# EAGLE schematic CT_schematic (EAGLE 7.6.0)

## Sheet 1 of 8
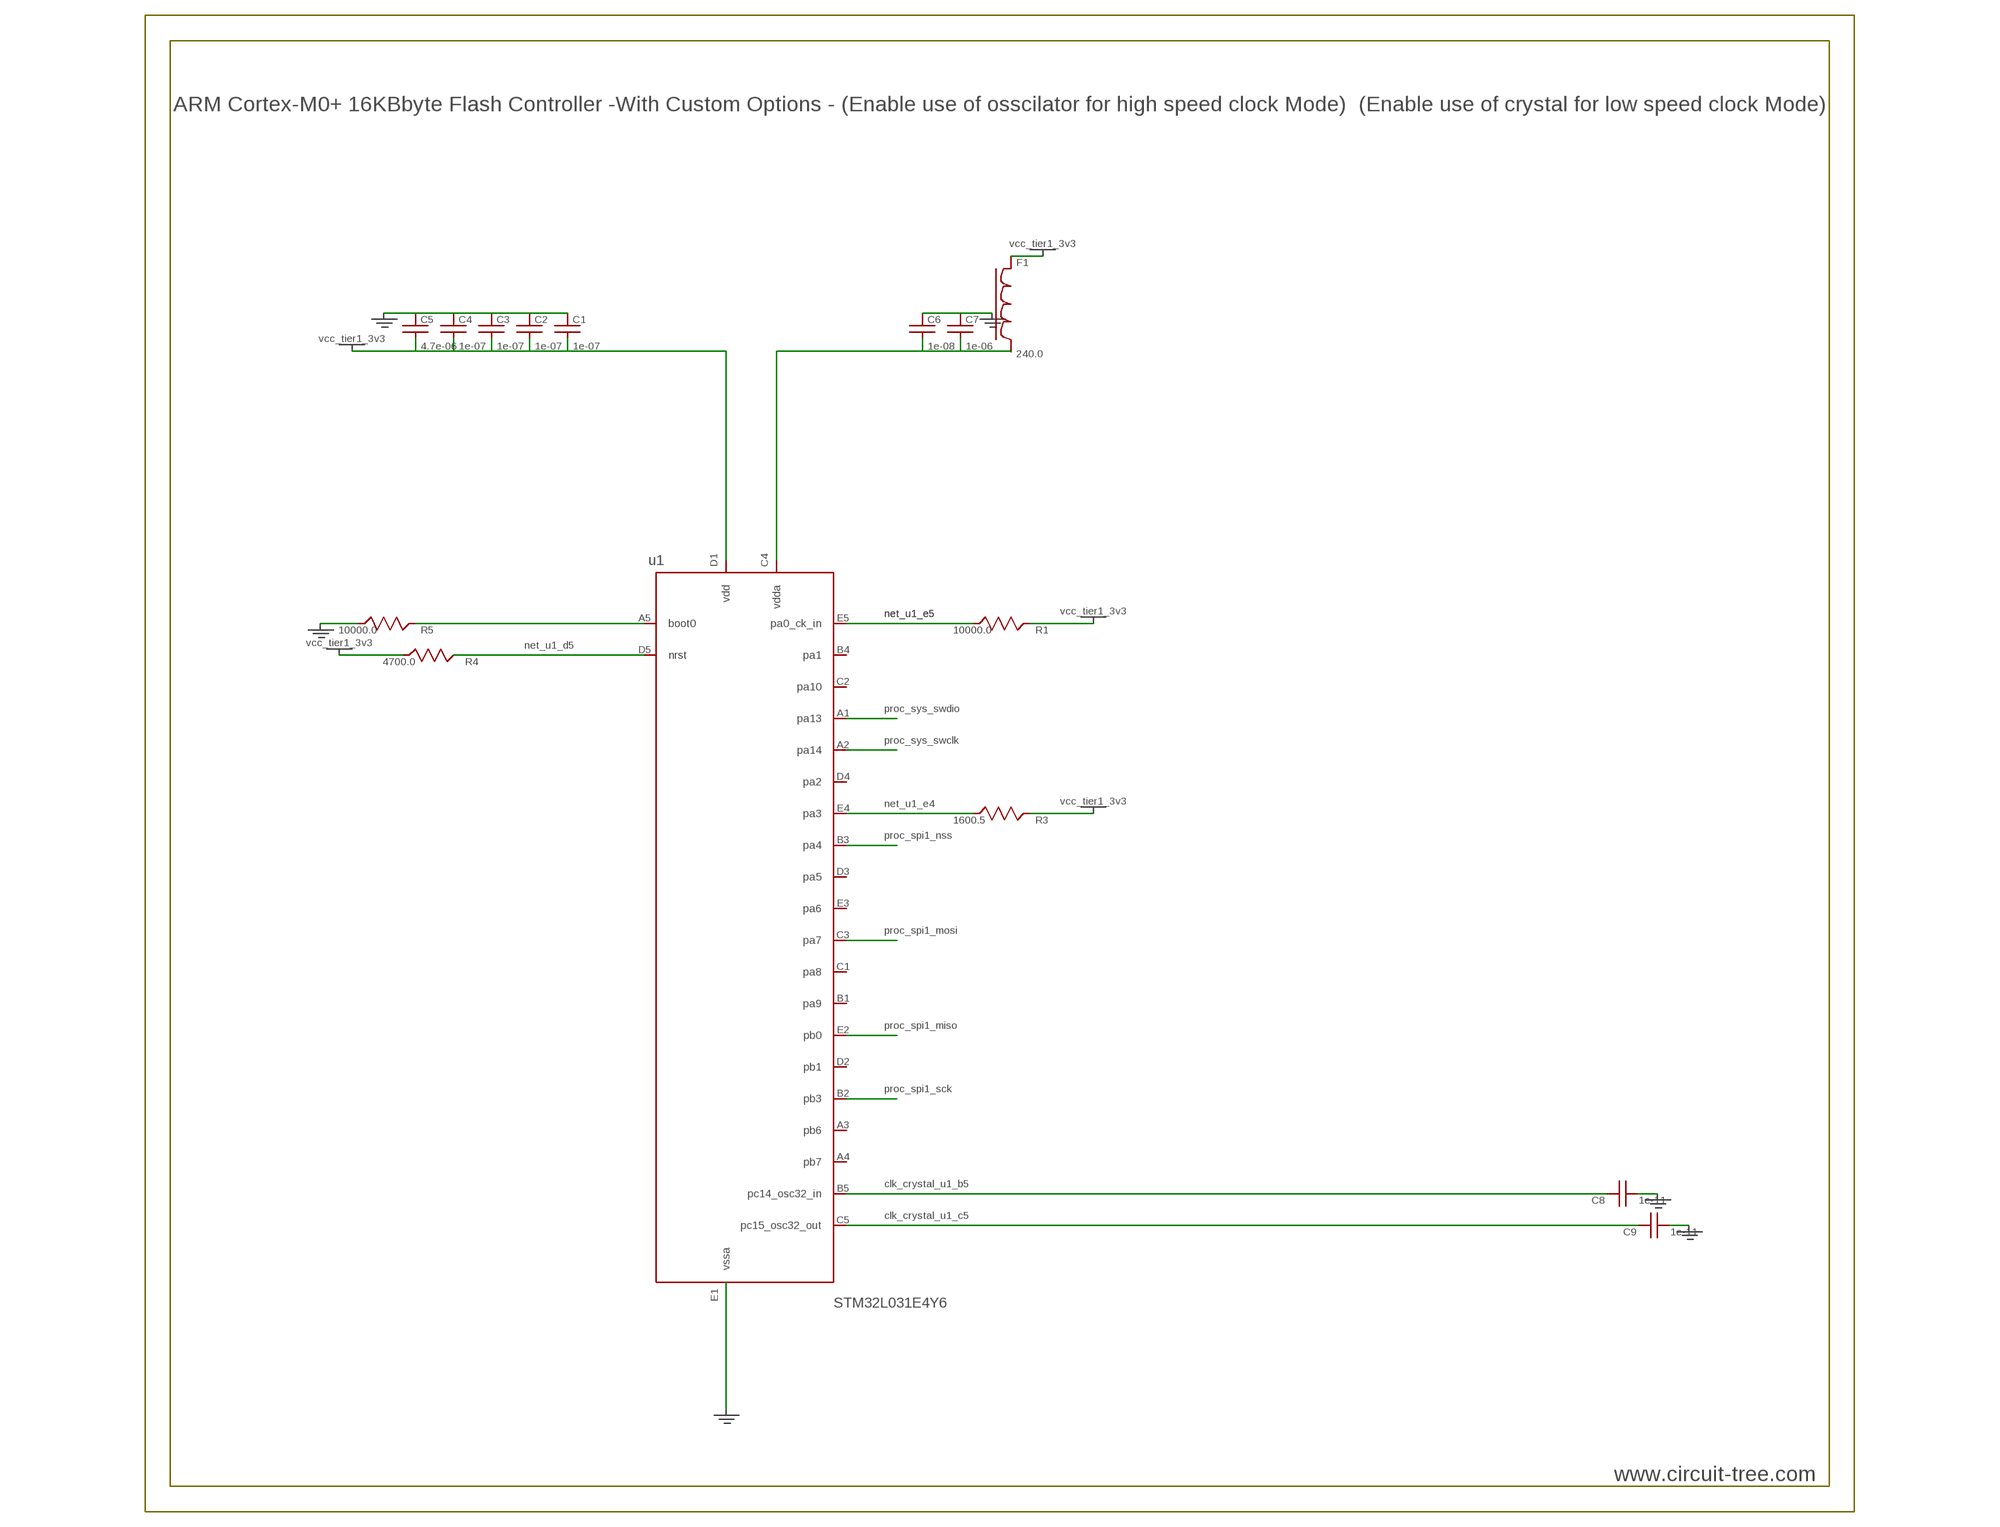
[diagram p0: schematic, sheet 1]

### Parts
C1  1e-07  06035C104K4Z2A  [C0603]
C2  1e-07  06035C104K4Z2A  [C0603]
C3  1e-07  06035C104K4Z2A  [C0603]
C4  1e-07  06035C104K4Z2A  [C0603]
C5  4.7e-06  GRM188R6YA475KE15D  [C0603]
C6  1e-08  06035C103K4Z2A  [C0603]
C7  1e-06  c0603c105k3ractu  [C0603]
C8  1e-11  C0402C100K3GACTU  [C0402]
C9  1e-11  C0402C100K3GACTU  [C0402]
F1  240.0  z0603c241asmst  [L0603]
R1  10000.0  RC0603JR-0710KL  [R0603]
R3  1600.5  R3  [R0603]
R4  4700.0  RC0603JR-074K7L  [R0603]
R5  10000.0  RC0603JR-0710KL  [R0603]
u1  STM32L031E4Y6  [WLCSP25]

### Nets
clk_crystal_u1_b5: C8.1 u1.B5(pc14_osc32_in) ; also sheet 4
clk_crystal_u1_c5: C9.1 u1.C5(pc15_osc32_out) ; also sheet 4
gnd: C1.2 C2.2 C3.2 C4.2 C5.2 C6.2 C7.2 C8.2 C9.2 R5.2 u1.E1(vssa) ; also sheet 2,3,4,5,6,7,8
net_u1_a5: R5.1 u1.A5(boot0)
net_u1_c4: C6.1 C7.1 F1.1 u1.C4(vdda)
net_u1_d5: R4.1 u1.D5(nrst) ; also sheet 8
net_u1_e4: R3.1 u1.E4(pa3) ; also sheet 8
net_u1_e5: R1.1 u1.E5(pa0_ck_in) ; also sheet 4,8
proc_spi1_miso: u1.E2(pb0) ; also sheet 3
proc_spi1_mosi: u1.C3(pa7) ; also sheet 3
proc_spi1_nss: u1.B3(pa4) ; also sheet 3
proc_spi1_sck: u1.B2(pb3) ; also sheet 3
proc_sys_swclk: u1.A2(pa14) ; also sheet 2
proc_sys_swdio: u1.A1(pa13) ; also sheet 2
vcc_tier1_3v3: C1.1 C2.1 C3.1 C4.1 C5.1 F1.2 R1.2 R3.2 R4.2 u1.D1(vdd) ; also sheet 2,3,4,5,6,8
Unconnected: u1.A3(pb6) u1.A4(pb7) u1.B1(pa9) u1.B4(pa1) u1.C1(pa8) u1.C2(pa10) u1.D2(pb1) u1.D3(pa5) u1.D4(pa2) u1.E3(pa6)

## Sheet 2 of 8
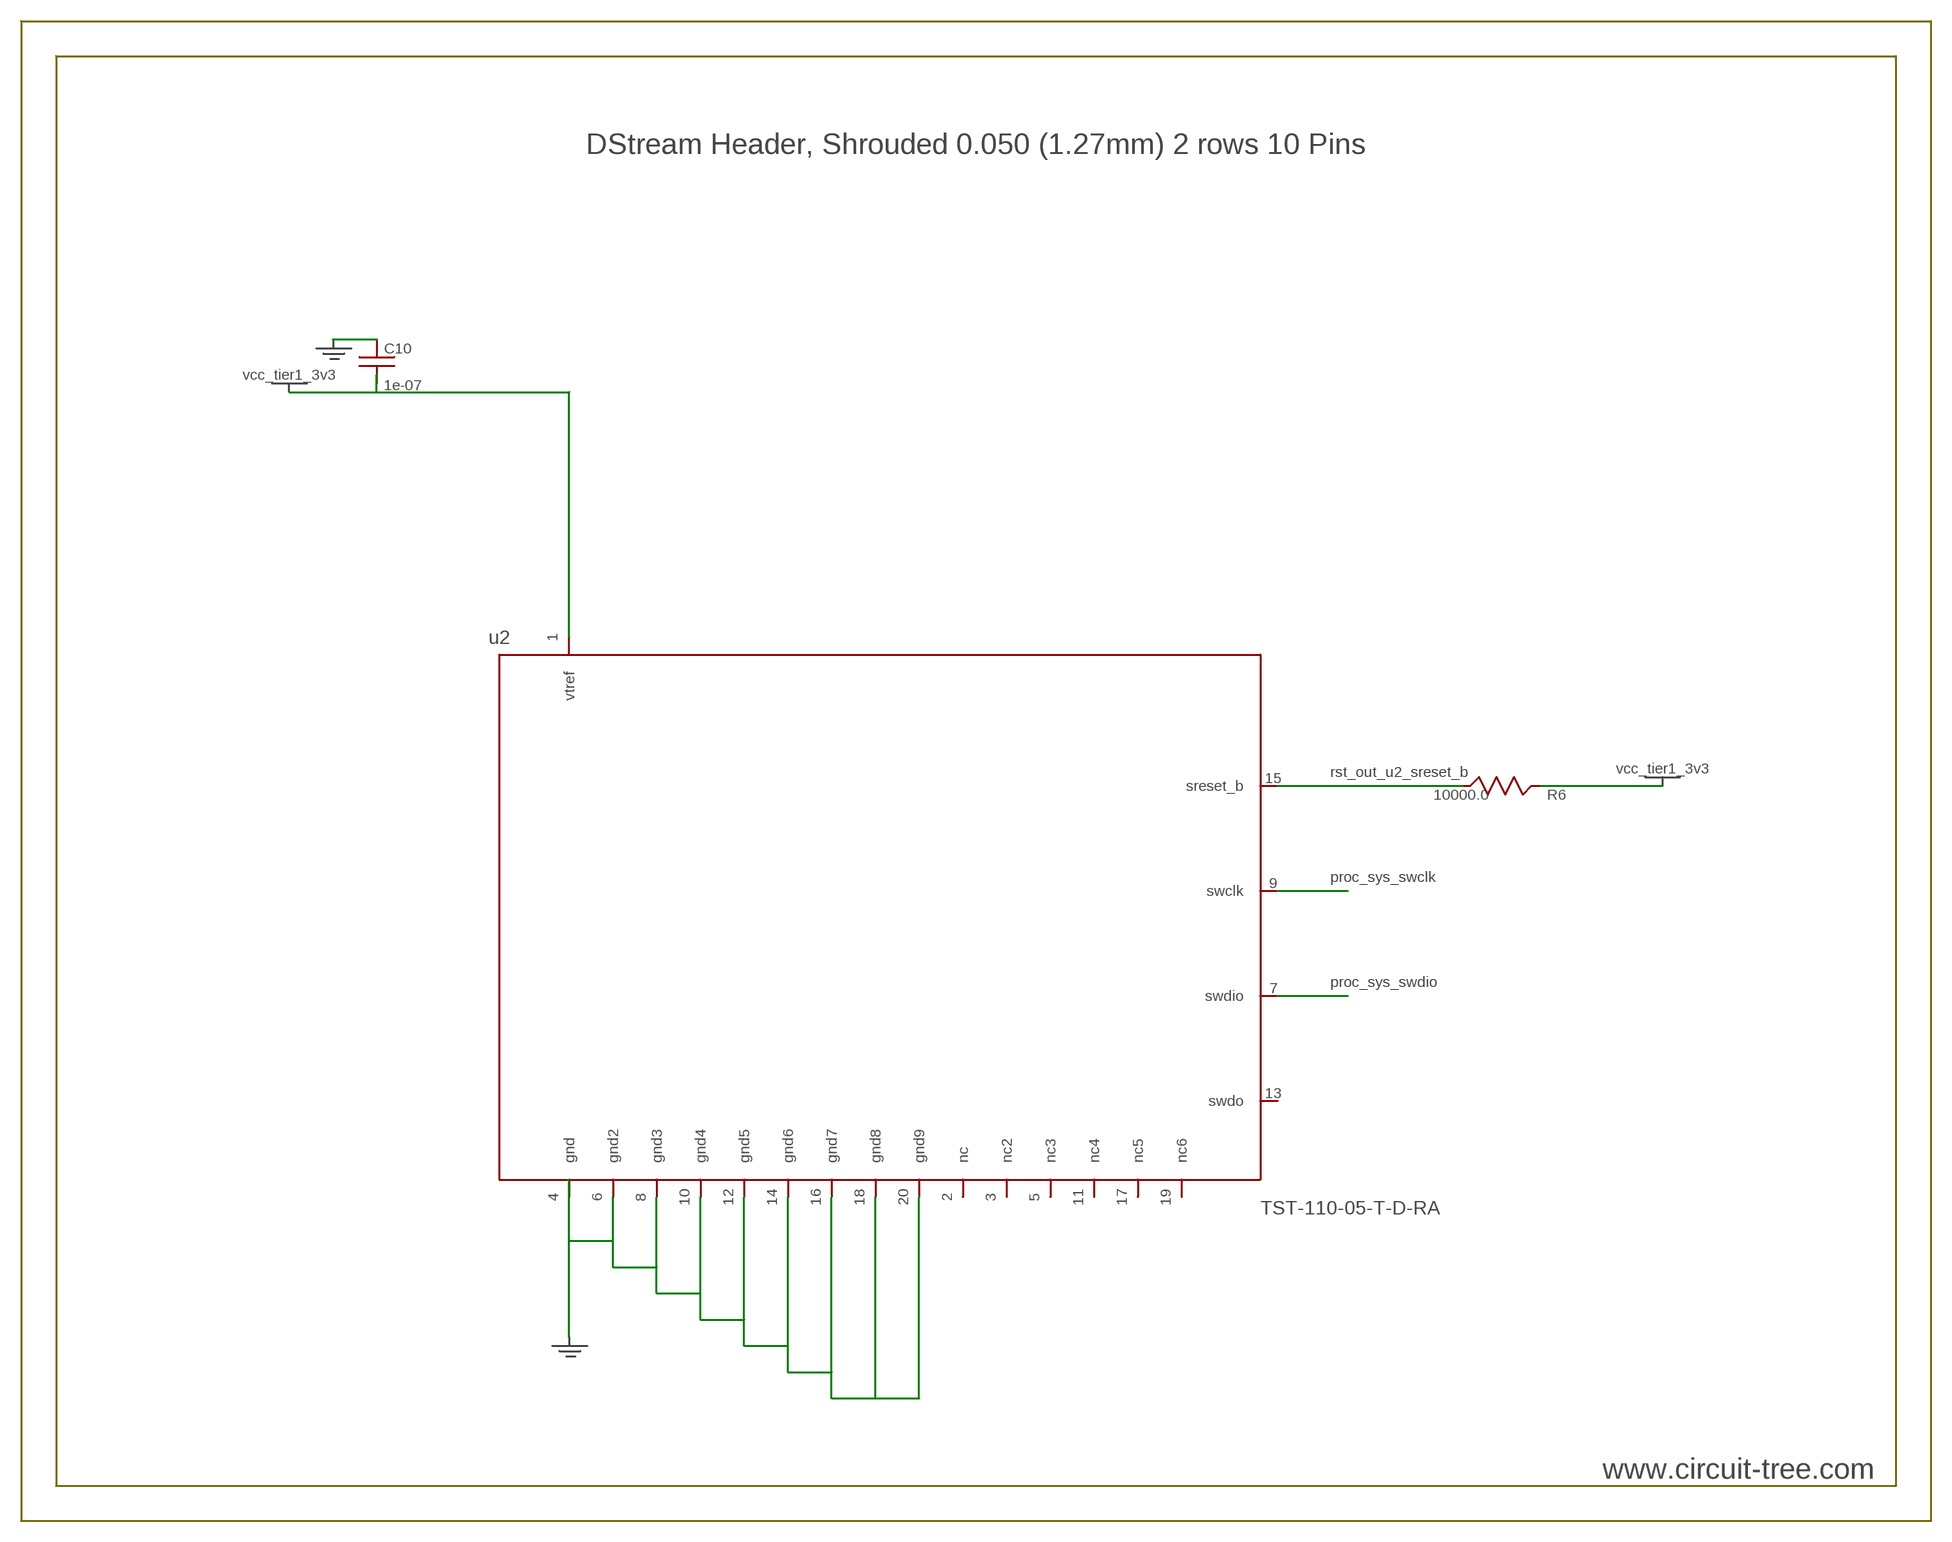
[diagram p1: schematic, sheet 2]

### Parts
C10  1e-07  c0402c104k3ractu  [C0402]
R6  10000.0  RC0603JR-0710KL  [R0603]
u2  TST-110-05-T-D-RA  [TST-110-05-T-D-RA]

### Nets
gnd: C10.2 u2.4(gnd) u2.6(gnd2) u2.8(gnd3) u2.10(gnd4) u2.12(gnd5) u2.14(gnd6) u2.16(gnd7) u2.18(gnd8) u2.20(gnd9) ; also sheet 1,3,4,5,6,7,8
proc_sys_swclk: u2.9(swclk) ; also sheet 1
proc_sys_swdio: u2.7(swdio) ; also sheet 1
rst_out_u2_sreset_b: R6.1 u2.15(sreset_b) ; also sheet 8
vcc_tier1_3v3: C10.1 R6.2 u2.1(vtref) ; also sheet 1,3,4,5,6,8
Unconnected: u2.2(nc) u2.3(nc2) u2.5(nc3) u2.11(nc4) u2.13(swdo) u2.17(nc5) u2.19(nc6)

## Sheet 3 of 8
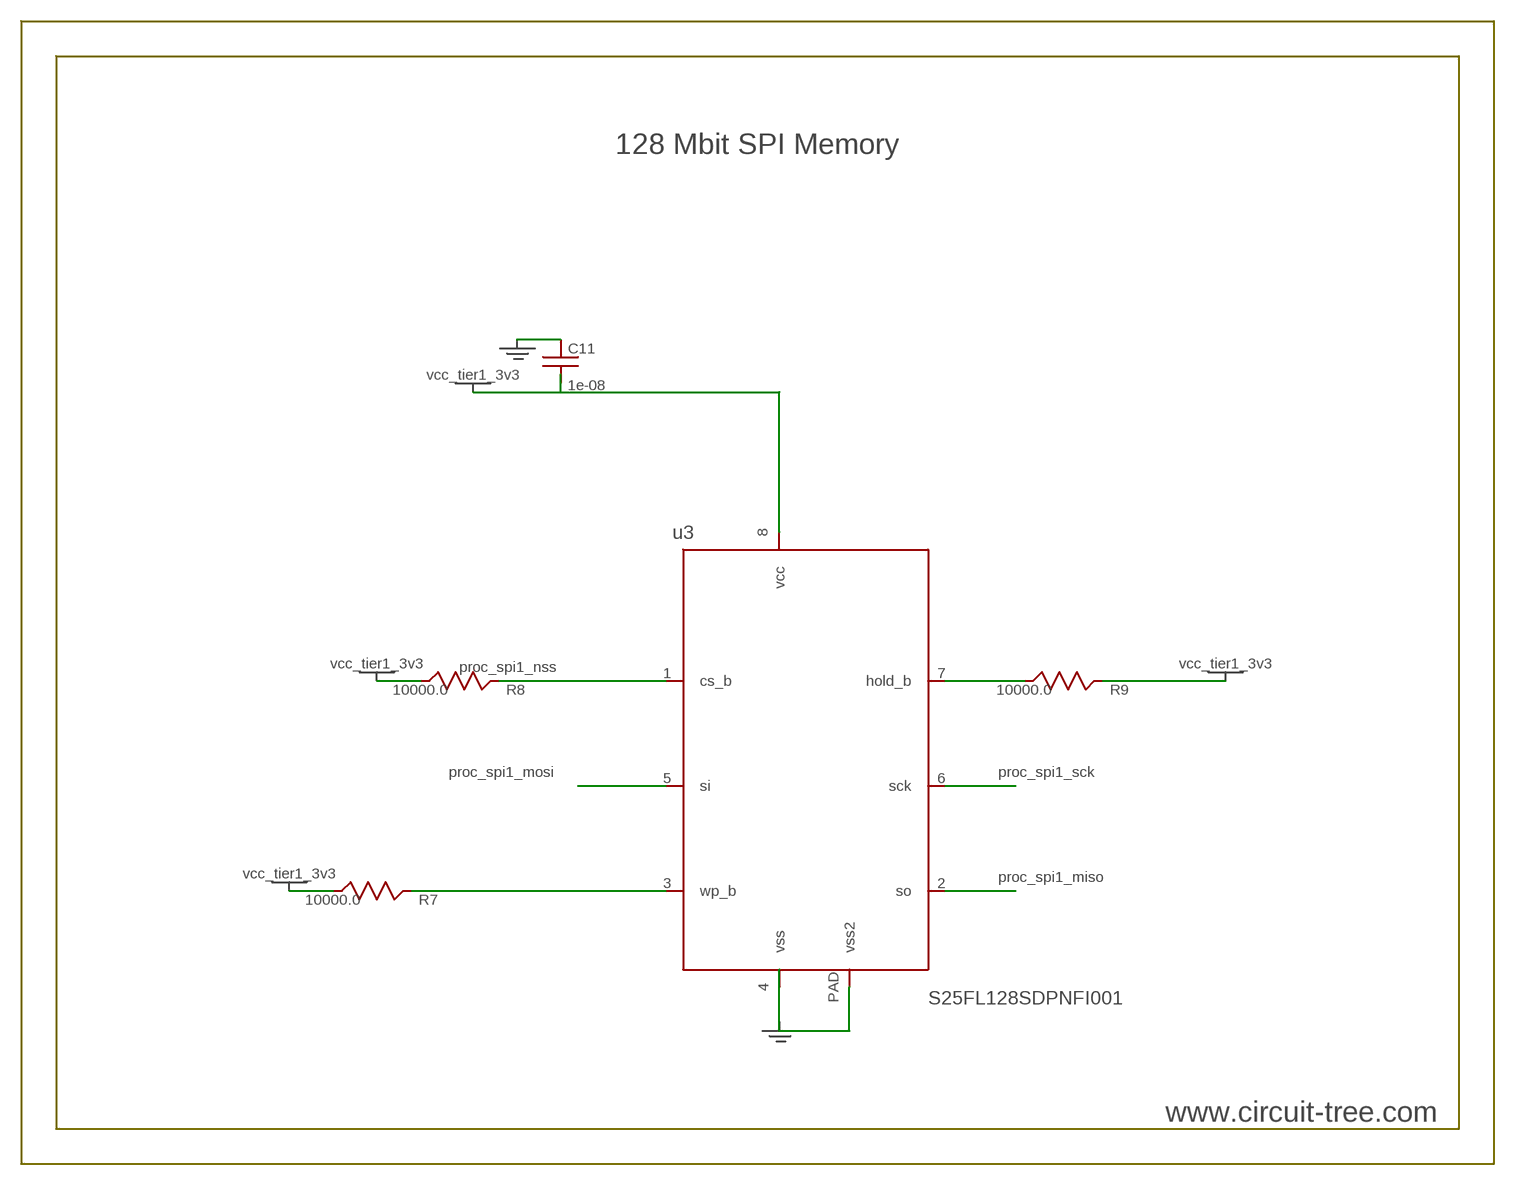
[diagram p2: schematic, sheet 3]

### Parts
C11  1e-08  c0402c103k3rac  [C0402]
R7  10000.0  RC0603JR-0710KL  [R0603]
R8  10000.0  RC0603JR-0710KL  [R0603]
R9  10000.0  RC0603JR-0710KL  [R0603]
u3  S25FL128SDPNFI001  [WNG008]

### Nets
gnd: C11.2 u3.4(vss) u3.PAD(vss2) ; also sheet 1,2,4,5,6,7,8
net_u3_3: R7.1 u3.3(wp_b)
net_u3_7: R9.1 u3.7(hold_b)
proc_spi1_miso: u3.2(so) ; also sheet 1
proc_spi1_mosi: u3.5(si) ; also sheet 1
proc_spi1_nss: R8.1 u3.1(cs_b) ; also sheet 1
proc_spi1_sck: u3.6(sck) ; also sheet 1
vcc_tier1_3v3: C11.1 R7.2 R8.2 R9.2 u3.8(vcc) ; also sheet 1,2,4,5,6,8

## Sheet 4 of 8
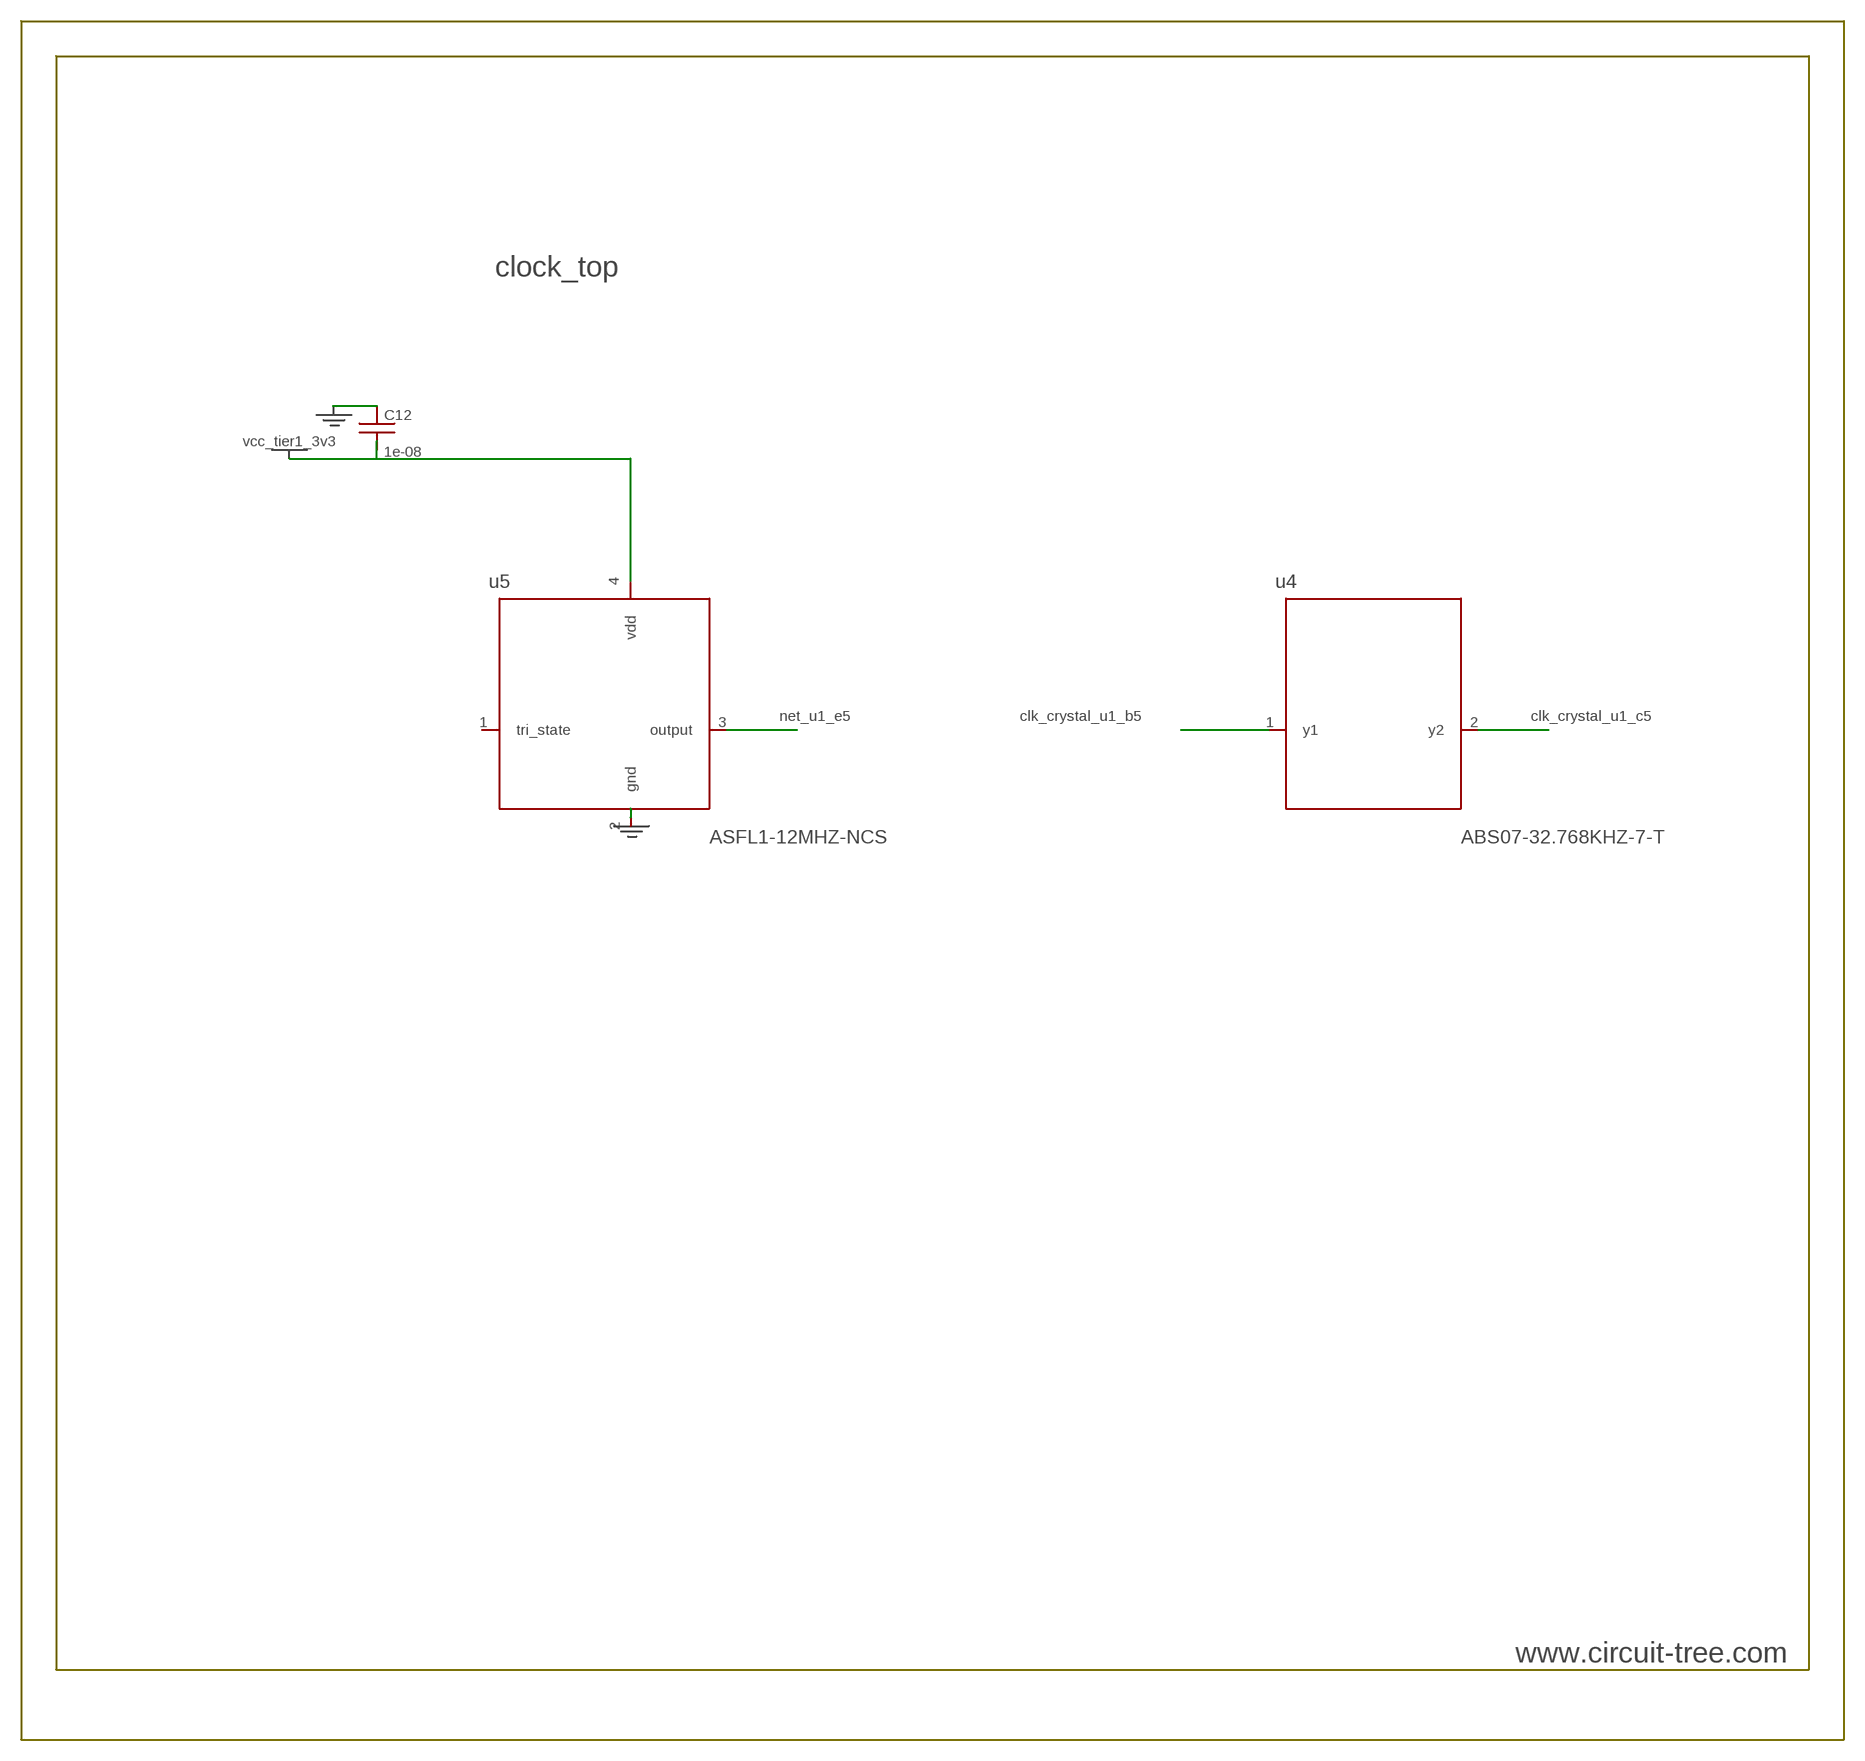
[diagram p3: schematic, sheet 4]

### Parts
C12  1e-08  c0402c103k3rac  [C0402]
u4  ABS07-32.768KHZ-7-T  [ABS07-32.768KHZ-7-T]
u5  ASFL1-12MHZ-NCS  [ASFL1]

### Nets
clk_crystal_u1_b5: u4.1(y1) ; also sheet 1
clk_crystal_u1_c5: u4.2(y2) ; also sheet 1
gnd: C12.2 u5.2(gnd) ; also sheet 1,2,3,5,6,7,8
net_u1_e5: u5.3(output) ; also sheet 1,8
vcc_tier1_3v3: C12.1 u5.4(vdd) ; also sheet 1,2,3,5,6,8
Unconnected: u5.1(tri_state)

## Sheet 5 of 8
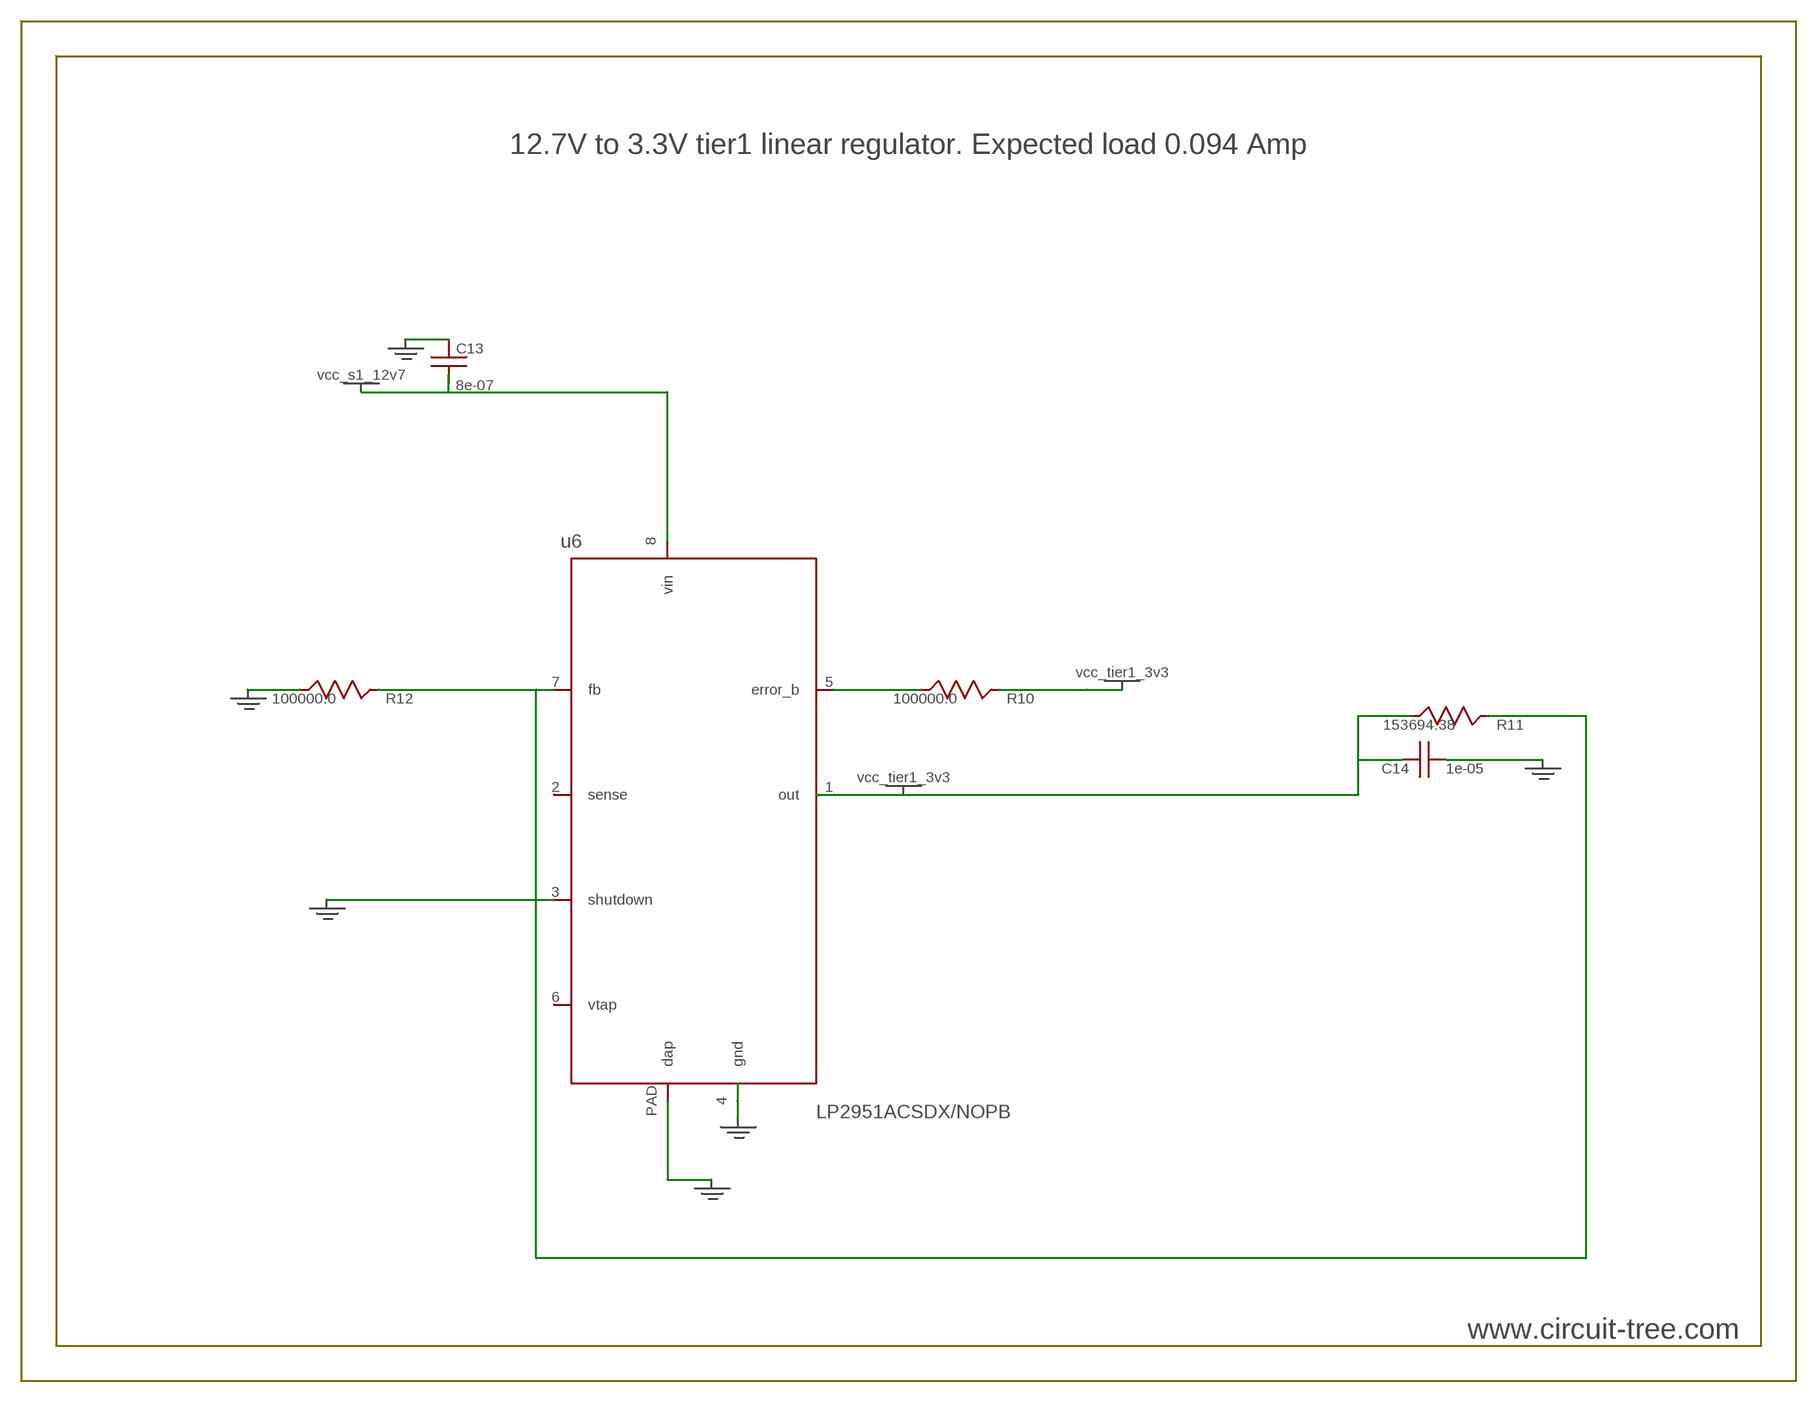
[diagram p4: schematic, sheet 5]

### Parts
C13  8e-07  C13  [R0603]
C14  1e-05  grm32DR61E106MA12L  [C1210]
R10  100000.0  RC0603JR-07100KL  [R0603]
R11  153694.38  R11  [R0603]
R12  100000.0  RC0603JR-07100KL  [R0603]
u6  LP2951ACSDX/NOPB  [WSON-8]

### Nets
gnd: C13.2 C14.2 R12.2 u6.3(shutdown) u6.4(gnd) u6.PAD(dap) ; also sheet 1,2,3,4,6,7,8
net_u6_5: R10.1 u6.5(error_b)
net_u6_7: R11.2 R12.1 u6.7(fb)
vcc_s1_12v7: C13.1 u6.8(vin) ; also sheet 7
vcc_tier1_3v3: c14.1 C14.1 r10.2 R10.2 r11.1 R11.1 u6.1(out) ; also sheet 1,2,3,4,6,8
Unconnected: u6.2(sense) u6.6(vtap)

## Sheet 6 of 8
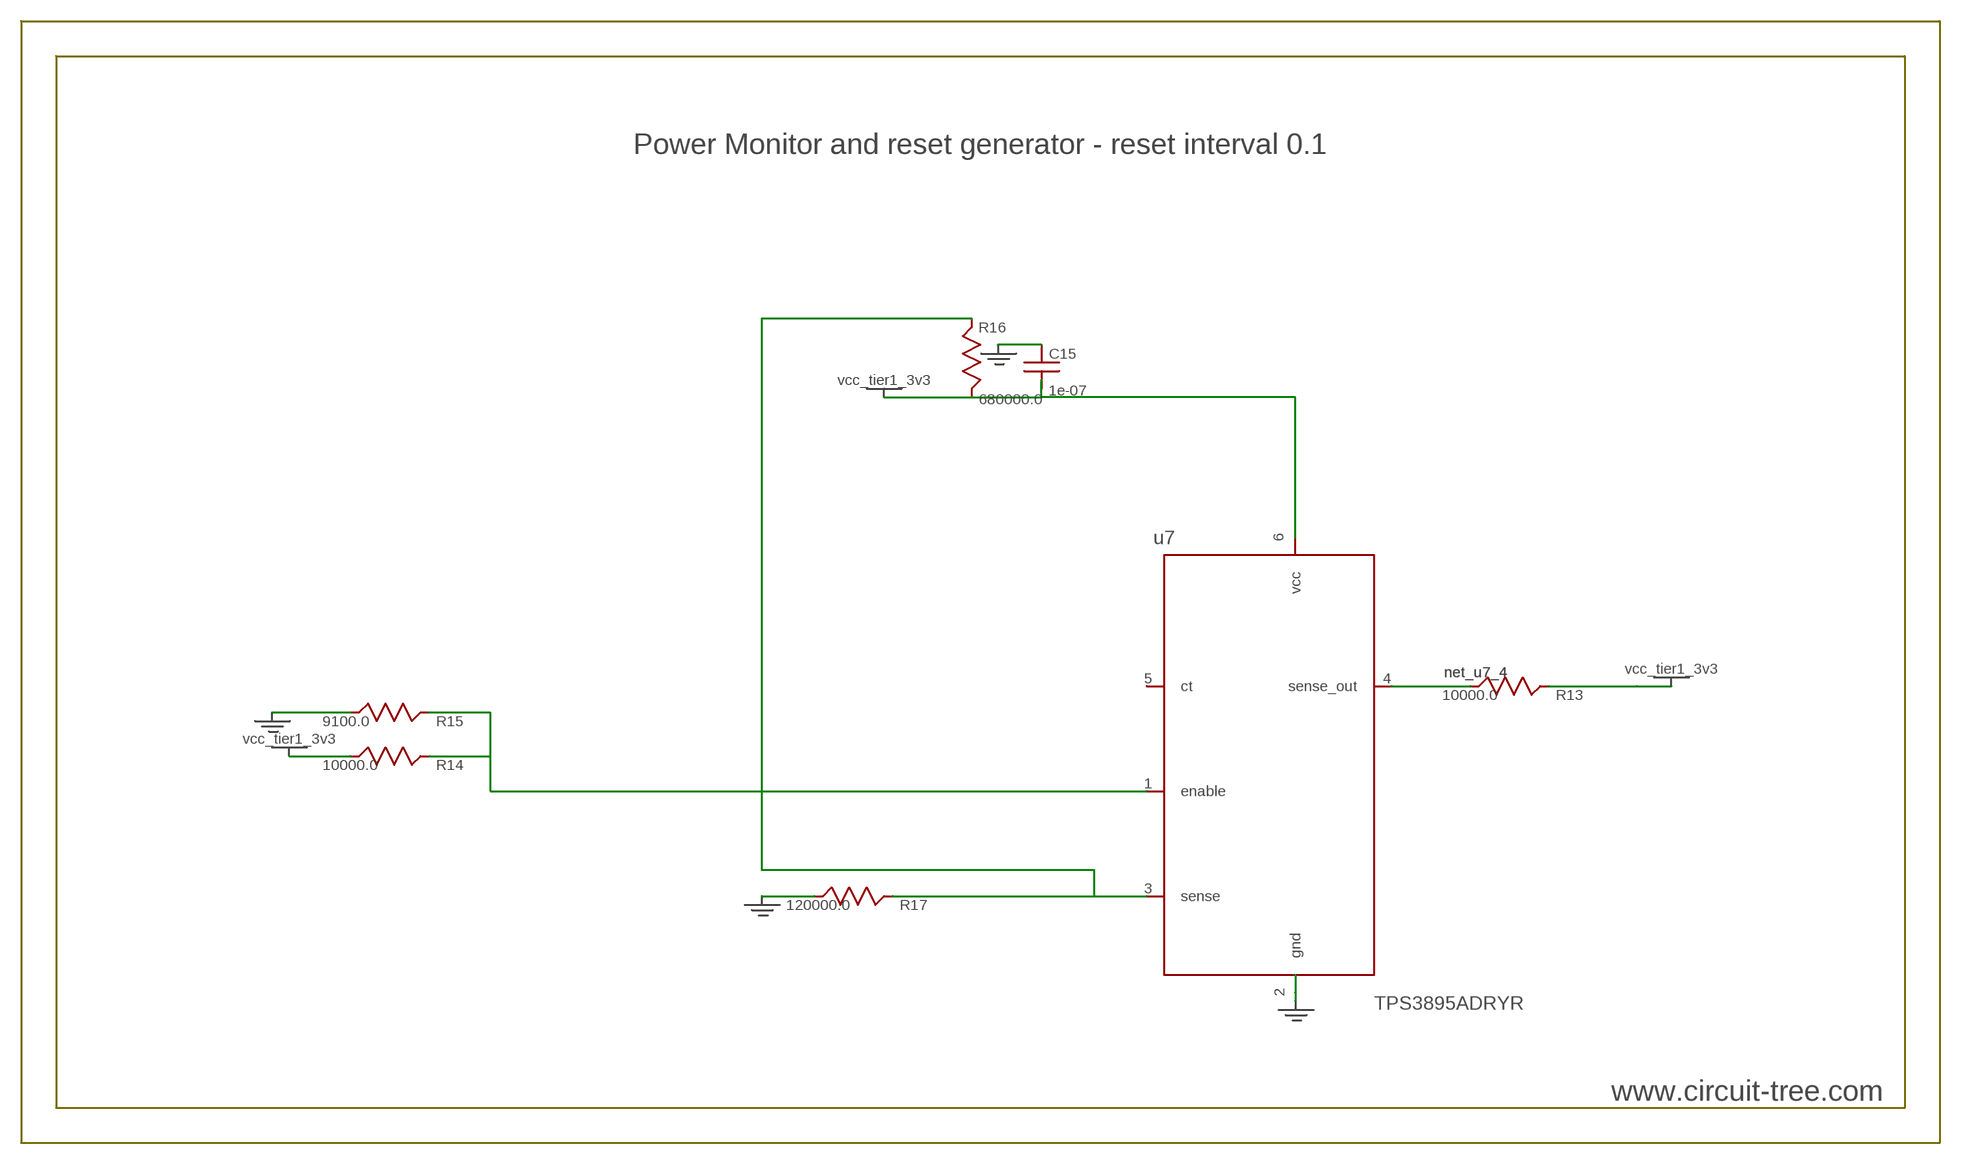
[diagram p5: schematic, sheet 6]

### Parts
C15  1e-07  c0402c104k3ractu  [C0402]
R13  10000.0  RC0603JR-0710KL  [R0603]
R14  10000.0  RC0603JR-0710KL  [R0603]
R15  9100.0  RC0603JR-079K1L  [R0603]
R16  680000.0  RC0603JR-07680KL  [R0603]
R17  120000.0  RC0603JR-07120KL  [R0603]
u7  TPS3895ADRYR  [SON-6]

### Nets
gnd: C15.2 R15.2 R17.2 u7.2(gnd) ; also sheet 1,2,3,4,5,7,8
net_u7_1: R14.1 R15.1 u7.1(enable)
net_u7_3: R16.2 R17.1 u7.3(sense)
net_u7_4: R13.1 u7.4(sense_out) ; also sheet 8
vcc_tier1_3v3: C15.1 R13.2 R14.2 R16.1 u7.6(vcc) ; also sheet 1,2,3,4,5,8
Unconnected: u7.5(ct)

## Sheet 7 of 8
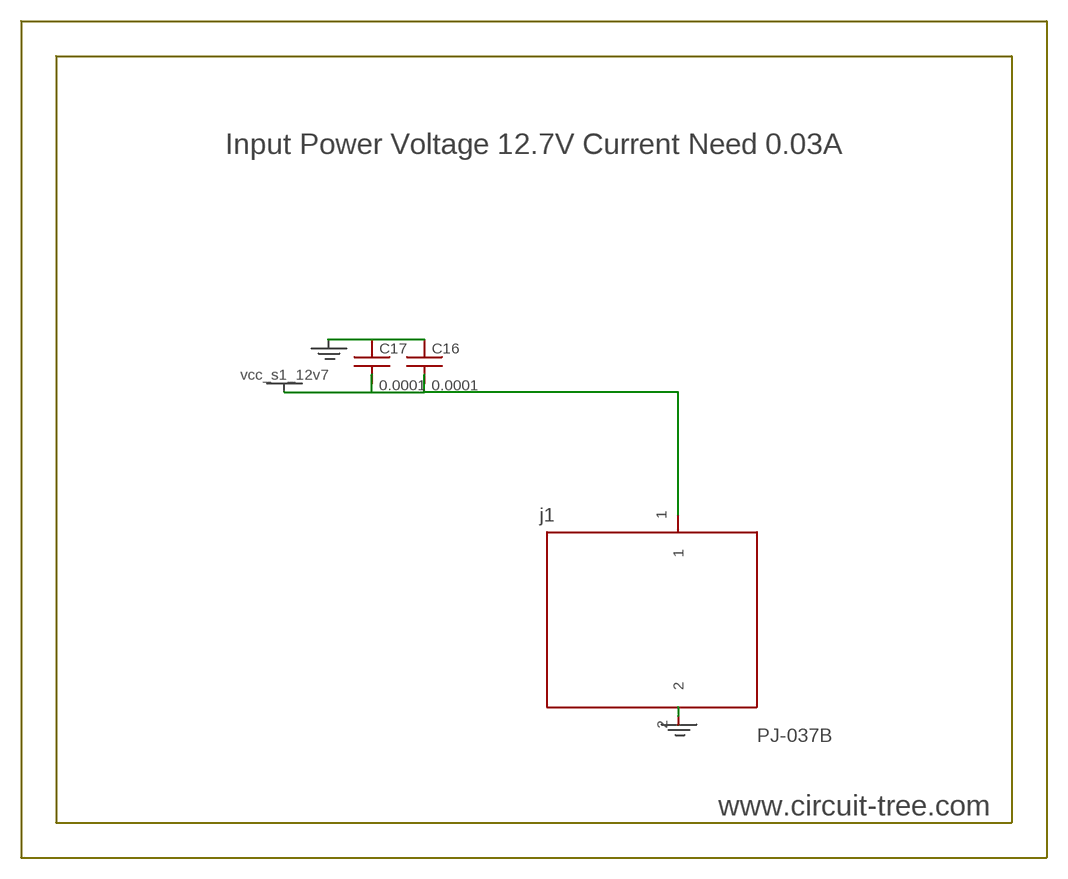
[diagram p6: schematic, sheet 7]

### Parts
C16  0.0001  edk107m035a9haa  [EXV-9H]
C17  0.0001  edk107m035a9haa  [EXV-9H]
j1  PJ-037B  [PJ-037B_PACKAGE]

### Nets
gnd: C16.2 C17.2 j1.2 ; also sheet 1,2,3,4,5,6,8
vcc_s1_12v7: C16.1 C17.1 j1.1 ; also sheet 5

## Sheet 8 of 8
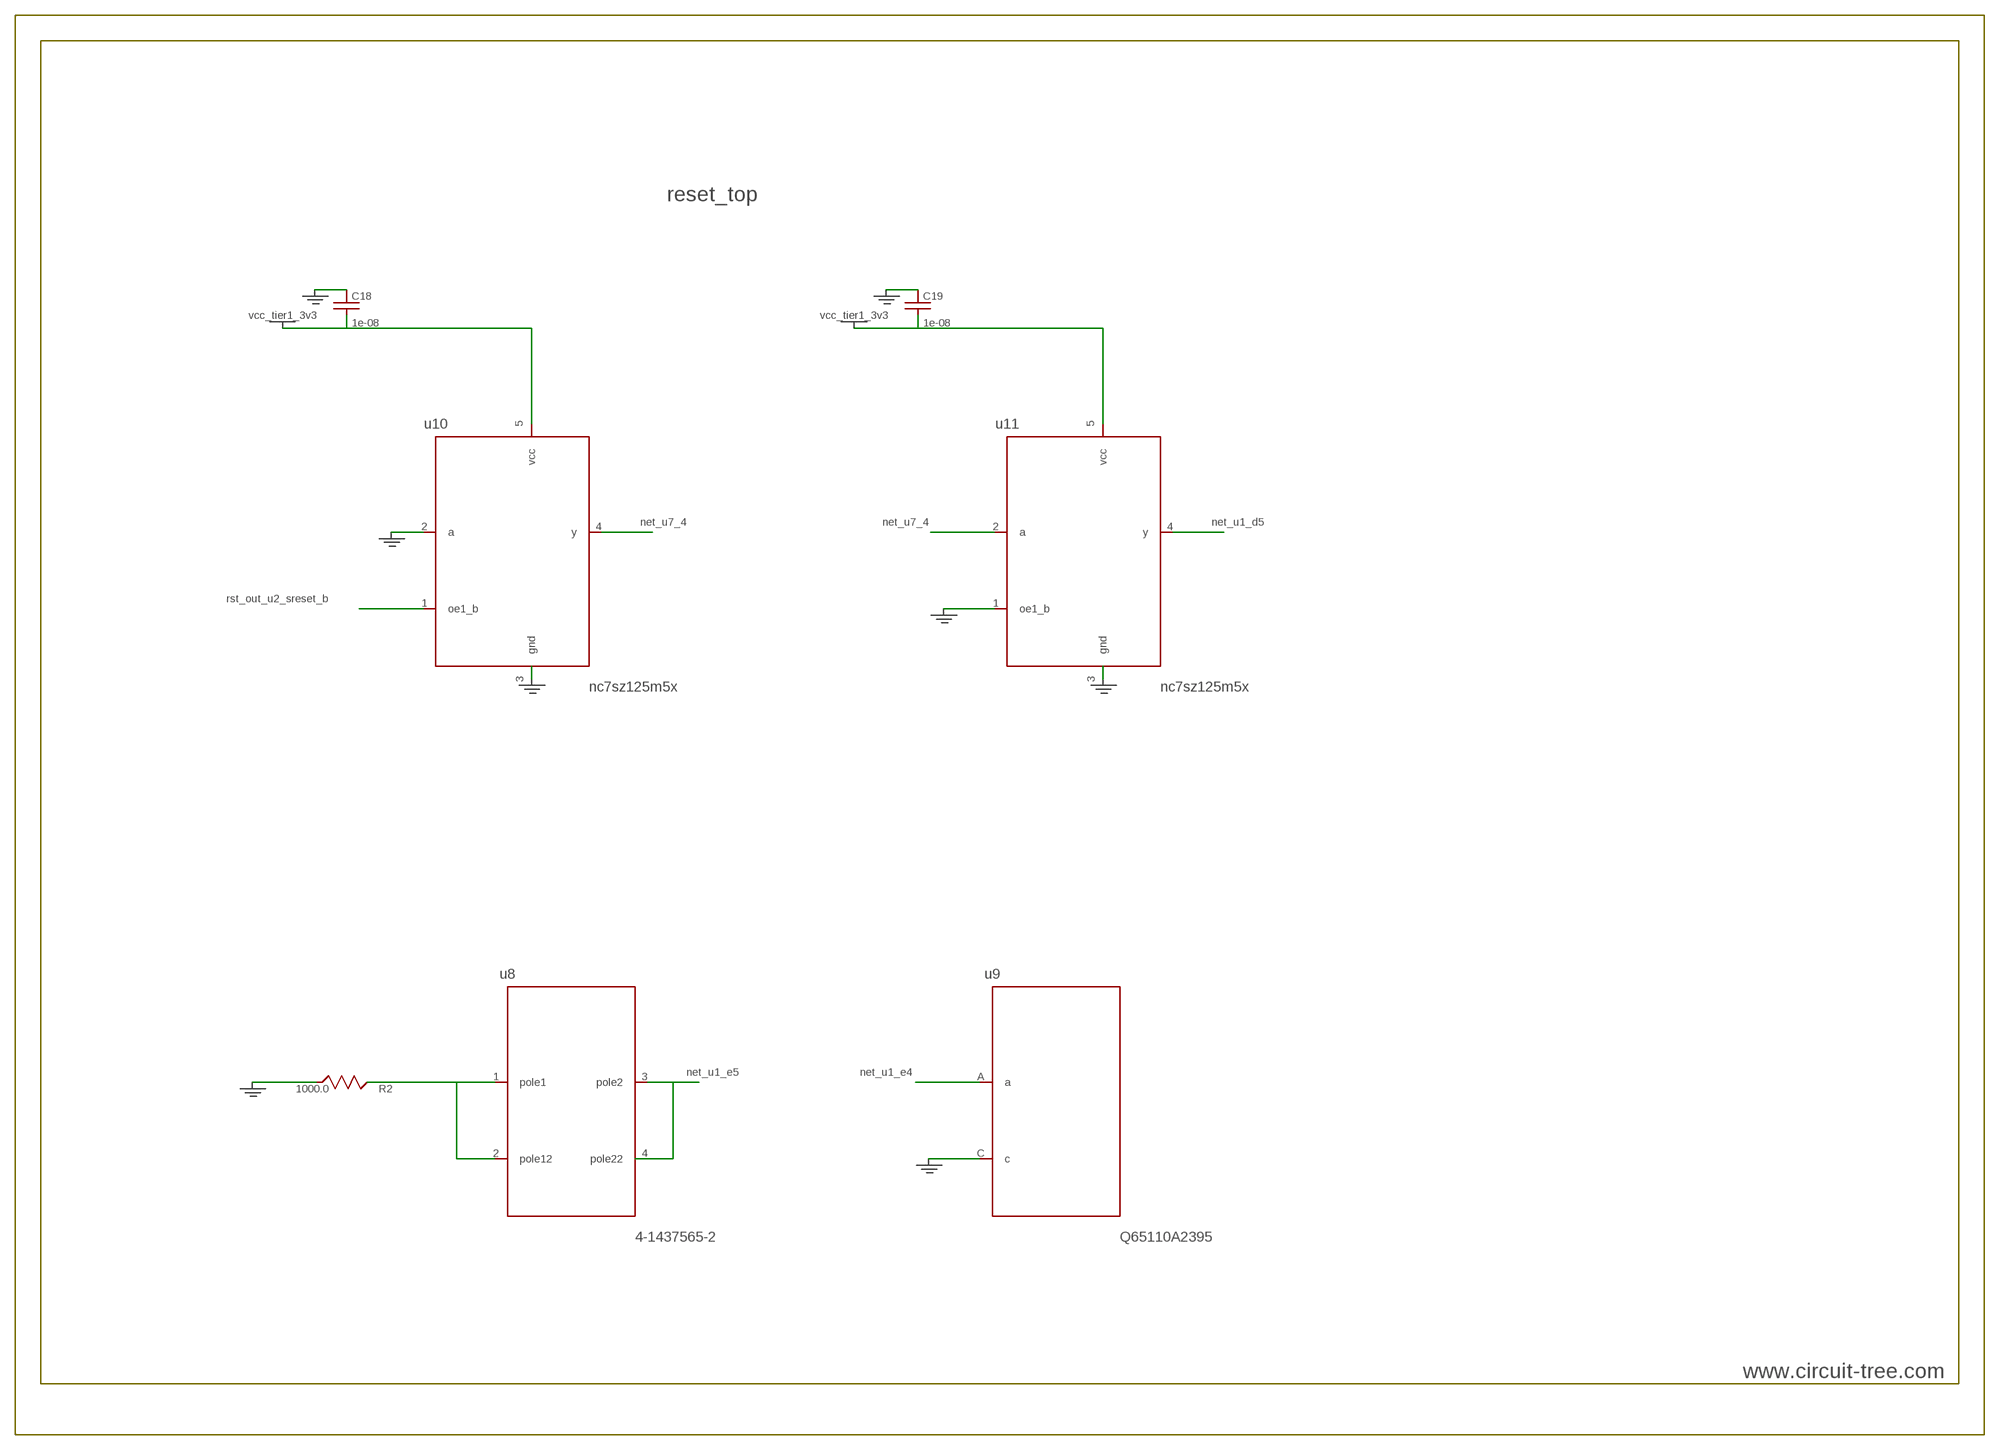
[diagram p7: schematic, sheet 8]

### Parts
C18  1e-08  c0402c103k3rac  [C0402]
C19  1e-08  c0402c103k3rac  [C0402]
R2  1000.0  RC0603JR-071KL  [R0603]
u8  4-1437565-2  [SW_4-1437565-2]
u9  Q65110A2395  [LGM67K-G1J2-24-Z]
u10  nc7sz125m5x  [nc7sz125m5x]
u11  nc7sz125m5x  [nc7sz125m5x]

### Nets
gnd: C18.2 C19.2 R2.2 u9.C(c) u10.2(a) u10.3(gnd) u11.1(oe1_b) u11.3(gnd) ; also sheet 1,2,3,4,5,6,7
net_u1_d5: u11.4(y) ; also sheet 1
net_u1_e4: u9.A(a) ; also sheet 1
net_u1_e5: u8.3(pole2) u8.4(pole22) ; also sheet 1,4
net_u7_4: u10.4(y) u11.2(a) ; also sheet 6
net_u8_1: R2.1 u8.1(pole1) u8.2(pole12)
rst_out_u2_sreset_b: u10.1(oe1_b) ; also sheet 2
vcc_tier1_3v3: C18.1 C19.1 u10.5(vcc) u11.5(vcc) ; also sheet 1,2,3,4,5,6

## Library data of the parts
C1-C4 = circuit_tree:06035C104K4Z2A: Capacitor
C5 = circuit_tree:GRM188R6YA475KE15D: Capacitor
C6 = circuit_tree:06035C103K4Z2A: Capacitor
C7 = circuit_tree:c0603c105k3ractu: Capacitor
C8 C9 = circuit_tree:C0402C100K3GACTU: Capacitor
C10 C15 = circuit_tree:c0402c104k3ractu: Capacitor
C11 C12 C18 C19 = circuit_tree:c0402c103k3rac: Capacitor
C13 = circuit_tree:C13: Capacitor
C14 = circuit_tree:grm32DR61E106MA12L: Capacitor
C16 C17 = circuit_tree:edk107m035a9haa: Capacitor
F1 = circuit_tree:z0603c241asmst: ferrite
j1 = circuit_tree:PJ-037B: IC
R1 R5-R9 R13 R14 = circuit_tree:RC0603JR-0710KL: Resistor
R2 = circuit_tree:RC0603JR-071KL: Resistor
R3 = circuit_tree:R3: Resistor
R4 = circuit_tree:RC0603JR-074K7L: Resistor
R10 R12 = circuit_tree:RC0603JR-07100KL: Resistor
R11 = circuit_tree:R11: Resistor
R15 = circuit_tree:RC0603JR-079K1L: Resistor
R16 = circuit_tree:RC0603JR-07680KL: Resistor
R17 = circuit_tree:RC0603JR-07120KL: Resistor
u1 = circuit_tree:STM32L031E4Y6: IC
u2 = circuit_tree:TST-110-05-T-D-RA: IC
u3 = circuit_tree:S25FL128SDPNFI001: IC
u4 = circuit_tree:ABS07-32.768KHZ-7-T: IC
u5 = circuit_tree:ASFL1-12MHZ-NCS: IC
u6 = circuit_tree:LP2951ACSDX/NOPB: IC
u7 = circuit_tree:TPS3895ADRYR: IC
u8 = circuit_tree:4-1437565-2: IC
u9 = circuit_tree:Q65110A2395: IC
u10 u11 = circuit_tree:nc7sz125m5x: IC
